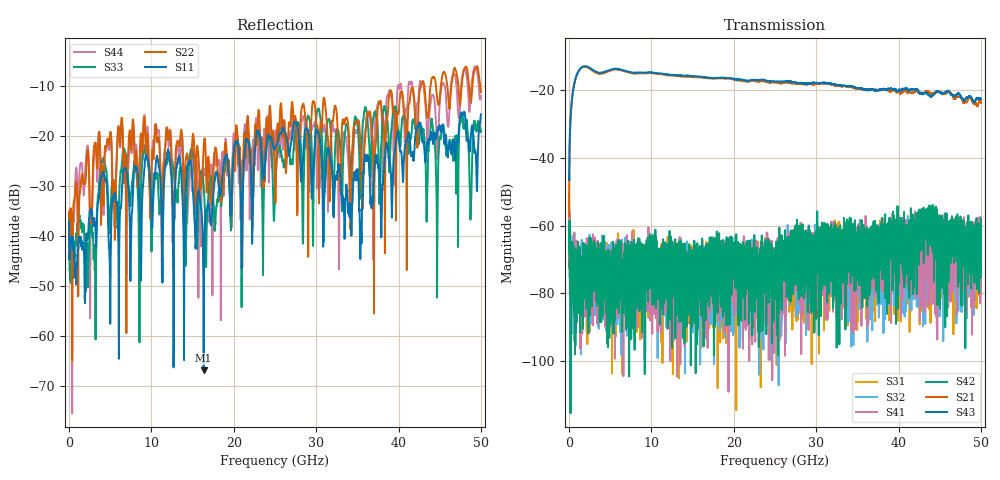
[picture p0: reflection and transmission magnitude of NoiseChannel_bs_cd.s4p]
!Keysight Technologies,N5245A,MY49151038,A.10.64.09
!Date: Tuesday, August 13, 2019 14:21:27
!Correction: S11(Full 4 Port(1,2,3,4))
!S12(Full 4 Port(1,2,3,4))
!S13(Full 4 Port(1,2,3,4))
!S14(Full 4 Port(1,2,3,4))
!S21(Full 4 Port(1,2,3,4))
!S22(Full 4 Port(1,2,3,4))
!S23(Full 4 Port(1,2,3,4))
!S24(Full 4 Port(1,2,3,4))
!S31(Full 4 Port(1,2,3,4))
!S32(Full 4 Port(1,2,3,4))
!S33(Full 4 Port(1,2,3,4))
!S34(Full 4 Port(1,2,3,4))
!S41(Full 4 Port(1,2,3,4))
!S42(Full 4 Port(1,2,3,4))
!S43(Full 4 Port(1,2,3,4))
!S44(Full 4 Port(1,2,3,4))
!S4P File: Measurements: <S11,S12,S13,S14>,
!<S21,S22,S23,S24>,
!<S31,S32,S33,S34>,
!<S41,S42,S43,S44>:
# Hz S  MA  R 50
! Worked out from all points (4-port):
!   5000 points, 10 MHz to 50 GHz, reference 50 ohm
!   strongest paths, dB at 10 MHz, 12.51 GHz, 25.01 GHz, 37.51 GHz, 50 GHz:
!     S43: -45.0, -15.5, -17.4, -20.0, -22.7
!     S21: -57.2, -15.7, -17.7, -20.1, -23.8
!     S42: -66.9, -67.8, -71.9, -62.0, -57.9
!     S41: -55.5, -73.1, -76.2, -65.8, -59.8
!     S32: -54.7, -77.2, -75.2, -68.3, -73.5
!     S31: -50.7, -75.8, -81.5, -78.1, -65.2
!   lowest |S11| = -66.9 dB at 16.34 GHz (marker M1), VSWR 1.00, Z = 50 - j0.0451 ohm
!   |S11| at or under -10 dB: start of sweep to end of sweep
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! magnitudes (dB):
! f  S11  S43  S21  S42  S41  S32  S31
! 10 MHz  -37.1  -45.0  -57.2  -66.9  -55.5  -54.7  -50.7
! 1.52 GHz  -42.0  -13.3  -13.5  -78.4  -71.1  -71.4  -66.7
! 12 GHz  -22.7  -15.4  -15.6  -69.0  -65.7  -69.3  -66.7
! 16.34 GHz  -66.9  -16.2  -16.4  -71.1  -79.8  -81.7  -73.9
! 22.94 GHz  -18.9  -17.0  -17.5  -71.1  -71.1  -86.1  -75.5
! 35.42 GHz  -39.2  -19.4  -19.7  -63.3  -70.7  -79.1  -68.0
! 50 GHz  -15.6  -22.7  -23.8  -57.9  -59.8  -73.5  -65.2
